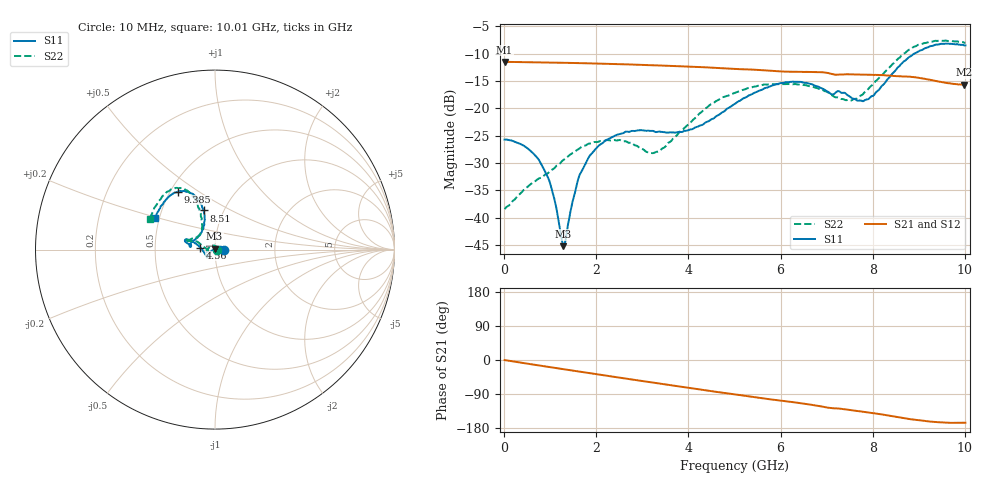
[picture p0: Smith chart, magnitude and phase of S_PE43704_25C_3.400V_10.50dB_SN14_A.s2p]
! Device ID: PE43704
! Dir: z:\PE43704\PE43704_Char_1_20130516\PE43704\AMB\3p400V\10p50dB
! Serial: 14
! Insertion: A
! Impedance: 50 ohm
! Temp: Amb
! VDD: 3.400V
! Attenuation Step: 10.50dB
! IDD: 1.140219e-01mA
#  Hz  S  RI  R  50
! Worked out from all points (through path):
!   401 points, 10 MHz to 10.01 GHz, reference 50 ohm
!   highest |S21| = -11.48 dB at 10 MHz (marker M1); lowest = -15.7 dB at 9.985 GHz (marker M2)
!   group delay of S21, straight-line fit = 47.7 ps
!   lowest |S11| = -45.2 dB at 1.285 GHz (marker M3), VSWR 1.01, Z = 49.8 + j0.498 ohm
!   |S11| at or under -10 dB: start of sweep to 8.895 GHz
!   |S22| runs from -38.4 to -7.6 dB; largest |S21 - S12| = 0.002
!   S11 on the Smith chart (normalised r, x): 10 MHz: 1.11, +0.00; 4.56 GHz: 0.85, +0.02; 8.51 GHz: 0.81, +0.37; 9.385 GHz: 0.55, +0.41; 10.01 GHz: 0.47, +0.20
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1e7  0.0518 0.00013  0.2668 -0.000981  0.2668 -0.000962  0.012 0.000361
4.35e8  0.0436 0.0124  0.2617 -0.0384  0.2621 -0.0385  0.0065 0.017
7.85e8  0.0274 0.0165  0.2548 -0.0679  0.2548 -0.0677  -0.00658 0.0221
1.035e9  0.0126 0.0128  0.2477 -0.0879  0.2476 -0.0877  -0.0189 0.0199
1.285e9  -0.00224 0.005  0.2384 -0.1072  0.2384 -0.1072  -0.0311 0.0131
1.56e9  -0.0178 -0.0059  0.2269 -0.1272  0.2269 -0.1272  -0.0411 0.00229
1.685e9  -0.0236 -0.0125  0.2208 -0.136  0.2209 -0.1358  -0.0445 -0.00308
1.91e9  -0.0321 -0.0222  0.2093 -0.1506  0.2094 -0.1505  -0.0467 -0.0115
2.26e9  -0.0391 -0.0347  0.1896 -0.1715  0.1897 -0.1714  -0.0471 -0.0202
3.36e9  -0.048 -0.0382  0.1162 -0.2181  0.1164 -0.2178  -0.0401 -0.00387
4.01e9  -0.062 -0.0135  0.0683 -0.231  0.0684 -0.2311  -0.0691 0.0203
4.56e9  -0.0809 0.011  0.0274 -0.2336  0.0278 -0.2336  -0.1032 0.0461
5.01e9  -0.1055 0.0318  -0.00329 -0.2296  -0.00296 -0.2298  -0.131 0.0463
5.96e9  -0.1582 0.0574  -0.0618 -0.2095  -0.0611 -0.2095  -0.1597 0.0464
6.685e9  -0.1611 0.0397  -0.1029 -0.1894  -0.1031 -0.1893  -0.15 0.0498
7.56e9  -0.1089 0.0572  -0.1391 -0.1502  -0.1392 -0.1506  -0.0807 0.0887
7.885e9  -0.0775 0.0928  -0.1517 -0.1354  -0.1514 -0.1358  -0.0712 0.1292
8.36e9  -0.0583 0.1833  -0.1674 -0.1085  -0.167 -0.1092  -0.0862 0.2206
8.51e9  -0.0625 0.2183  -0.1715 -0.0975  -0.1708 -0.0985  -0.0986 0.2562
9.385e9  -0.2071 0.3226  -0.1707 -0.0495  -0.1712 -0.049  -0.2512 0.3299
9.985e9  -0.327 0.1879  -0.1594 -0.0404  -0.1601 -0.04  -0.3571 0.1788
1.001e10  -0.3328 0.1777  -0.1598 -0.0411  -0.1605 -0.0408  -0.3605 0.1706
